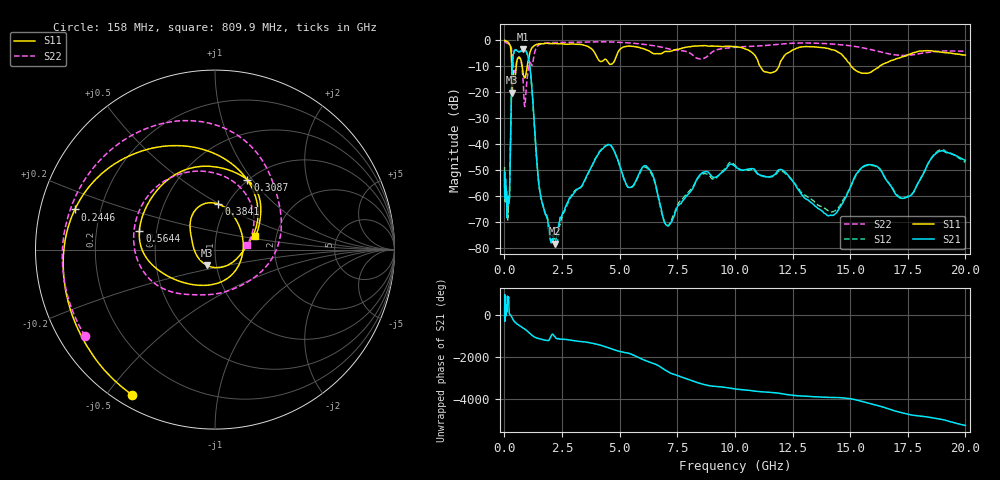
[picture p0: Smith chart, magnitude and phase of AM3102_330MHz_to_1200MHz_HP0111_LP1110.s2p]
! Date/Time: Tue, Sep 11, 2018 5:16 PM
! Network Analyzer: Agilent Technologies E8362B Rev: A.07.50.63
! Sweep from 0.010 to 20.000 GHz, 1601 Points, Sweep Type: LOG
! Power Supply: 4.949 V, 0.001 A
# Hz S DB R 50
!freq MagS11 AngS11 MagS21 AngS21 MagS12 AngS12 MagS22 AngS22
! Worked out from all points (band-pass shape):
!   1601 points, 10 MHz to 20 GHz, reference 50 ohm
!   highest |S21| = -3.42 dB at 821.5 MHz (marker M1); lowest = -78.5 dB at 2.196 GHz (marker M2)
!   |S21| within 3 dB of the highest: 372.5 MHz to 1.033 GHz (660.3 MHz wide, 94 % of centre)
!   lowest |S11| = -20.1 dB at 341.1 MHz (marker M3), VSWR 1.22, Z = 45 - j7.98 ohm
!   |S11| at or under -10 dB: 771.4 MHz to 989.4 MHz (218.1 MHz wide, 24.8 % of centre); 11.09 GHz to 11.91 GHz (819.8 MHz wide, 7.13 % of centre); 15.04 GHz to 16.28 GHz (1.235 GHz wide, 7.88 % of centre)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
!   |S22| runs from -25.5 to -0.3 dB; largest |S21 - S12| = 0.012
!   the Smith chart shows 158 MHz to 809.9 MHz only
!   S11 on the Smith chart (normalised r, x): 158 MHz: 0.05, -0.58; 244.6 MHz: 0.11, +0.14; 308.7 MHz: 1.00, +0.94; 384.1 MHz: 0.91, +0.49; 564.4 MHz: 0.40, +0.10; 809.9 MHz: 1.56, +0.24
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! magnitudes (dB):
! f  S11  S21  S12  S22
! 10 MHz  0.0  -59.2  -48.9  -0.3
! 35.55 MHz  0.0  -59.8  -59.3  -0.6
! 126.4 MHz  -0.4  -67.4  -63.0  -1.1
! 158 MHz  -0.6  -60.5  -66.3  -1.2
! 244.6 MHz  -1.8  -50.5  -50.6  -1.7
! 308.7 MHz  -7.4  -19.6  -19.6  -3.3
! 341.1 MHz  -20.1  -9.9  -9.9  -5.9
! 384.1 MHz  -11.9  -5.7  -5.8  -9.4
! 447.2 MHz  -15.6  -3.8  -3.9  -12.3
! 564.4 MHz  -7.3  -4.1  -4.2  -7.1
! 809.9 MHz  -12.5  -3.4  -3.5  -15.0
! 821.5 MHz  -13.1  -3.4  -3.5  -16.7
! 1.119 GHz  -4.4  -11.2  -11.3  -8.4
! 1.59 GHz  -1.3  -60.7  -61.1  -1.3
! 2.196 GHz  -1.2  -78.5  -77.2  -0.8
! 4.373 GHz  -7.2  -40.9  -40.8  -0.5
! 5.652 GHz  -2.4  -55.2  -55.4  -1.1
! 6.245 GHz  -3.9  -49.3  -49.8  -1.7
! 7.134 GHz  -4.3  -71.5  -71.2  -3.3
! 10.09 GHz  -2.4  -49.2  -49.0  -2.5
! 14.07 GHz  -3.1  -67.7  -65.9  -1.3
! 20 GHz  -5.7  -46.3  -47.1  -4.2
